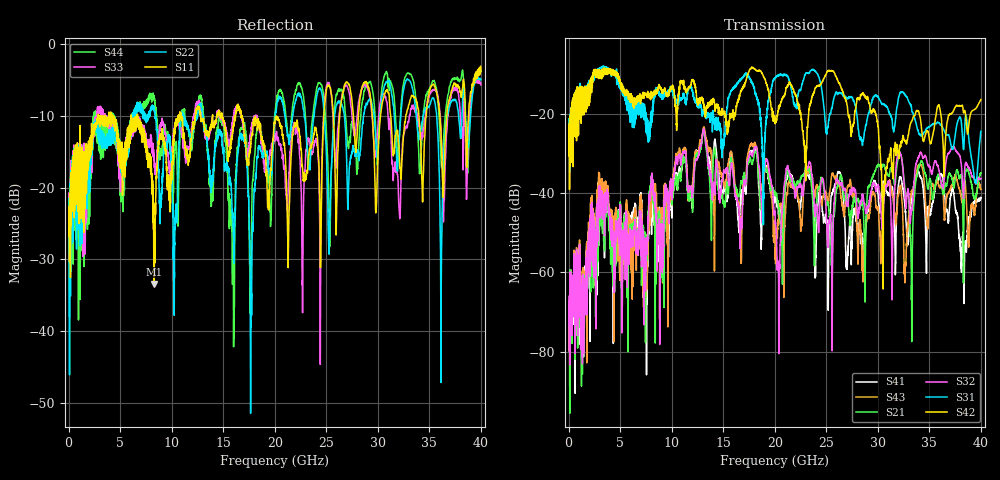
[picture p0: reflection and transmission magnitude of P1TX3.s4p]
!Agilent Technologies,N5245A,MY49151084,A.09.20.08
!Agilent N5245A: A.09.20.08
!Date: Thursday, March 01, 2012 11:57:10
!Correction: S11(Full 4 Port(1,2,3,4))
!S12(Full 4 Port(1,2,3,4))
!S13(Full 4 Port(1,2,3,4))
!S14(Full 4 Port(1,2,3,4))
!S21(Full 4 Port(1,2,3,4))
!S22(Full 4 Port(1,2,3,4))
!S23(Full 4 Port(1,2,3,4))
!S24(Full 4 Port(1,2,3,4))
!S31(Full 4 Port(1,2,3,4))
!S32(Full 4 Port(1,2,3,4))
!S33(Full 4 Port(1,2,3,4))
!S34(Full 4 Port(1,2,3,4))
!S41(Full 4 Port(1,2,3,4))
!S42(Full 4 Port(1,2,3,4))
!S43(Full 4 Port(1,2,3,4))
!S44(Full 4 Port(1,2,3,4))
!S4P File: Measurements: <S11,S12,S13,S14>,
!<S21,S22,S23,S24>,
!<S31,S32,S33,S34>,
!<S41,S42,S43,S44>:
# Hz S  dB  R 50
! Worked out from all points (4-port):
!   3996 points, 50 MHz to 40 GHz, reference 50 ohm
!   strongest paths, dB at 50 MHz, 10.04 GHz, 20.03 GHz, 30.02 GHz, 40 GHz:
!     S42: -26.9, -13.3, -22.2, -23.3, -16.4
!     S31: -25.3, -14.1, -11.1, -15.9, -24.4
!     S32: -66.0, -40.9, -45.2, -38.0, -36.3
!     S21: -70.0, -42.5, -39.7, -32.9, -35.0
!     S43: -69.0, -39.5, -56.7, -43.6, -39.1
!     S41: -68.4, -42.7, -41.0, -40.1, -41.2
!   lowest |S11| = -33.4 dB at 8.31 GHz (marker M1), VSWR 1.04, Z = 52.1 - j0.633 ohm
!   |S11| at or under -10 dB: start of sweep to 2.877 GHz; 6.682 GHz to 10.63 GHz (3.947 GHz wide, 45.6 % of centre); 16.82 GHz to 24.76 GHz (7.937 GHz wide, 38.2 % of centre)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
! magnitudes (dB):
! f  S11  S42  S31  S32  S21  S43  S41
! 50 MHz  -24.7  -26.9  -25.3  -66.0  -70.0  -69.0  -68.4
! 8.31 GHz  -33.4  -14.9  -16.0  -40.7  -43.9  -40.1  -45.0
! 13.1 GHz  -10.8  -17.5  -20.0  -23.9  -24.4  -23.5  -24.1
! 20.06 GHz  -10.2  -21.9  -11.0  -47.7  -40.6  -53.8  -41.9
! 25.6 GHz  -8.4  -9.3  -17.8  -58.8  -50.1  -35.4  -40.0
! 30.56 GHz  -7.5  -38.9  -17.7  -43.2  -32.8  -41.7  -37.4
! 40 GHz  -3.8  -16.4  -24.4  -36.3  -35.0  -39.1  -41.2
